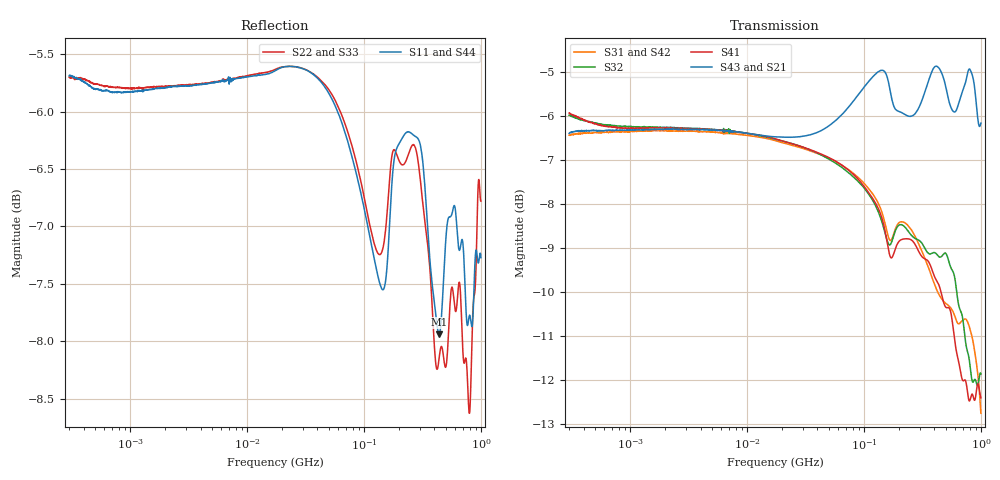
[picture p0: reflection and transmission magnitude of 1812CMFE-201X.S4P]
!s-Parameter Generated by FASTRON Sdn. Bhd.
!FASTRON P/N : 1812CMF/E-201X
!Keysight Technologies: E5071C_MY46733604_B.14.02
!Date: Mon Mar 09 11:25:32 2026
!Version  :Rev00  Mon Mar 09 11:25:32 2026
!Data & Calibration Information:
!Freq	S11:SOLT4(ON)	S12:SOLT4(ON)	S13:SOLT4(ON)	S14:SOLT4(ON)
!	S21:SOLT4(ON)	S22:SOLT4(ON)	S23:SOLT4(ON)	S24:SOLT4(ON)
!	S31:SOLT4(ON)	S32:SOLT4(ON)	S33:SOLT4(ON)	S34:SOLT4(ON)
!	S41:SOLT4(ON)	S42:SOLT4(ON)	S43:SOLT4(ON)	S44:SOLT4(ON)
!PortZ  Port1:50+j0  Port2:50+j0  Port3:50+j0  Port4:50+j0
!When reading reference impedance value at option line is always used.
! Remarks : This data is being provided solely for informational purposes.
# Hz S dB R 50
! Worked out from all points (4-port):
!   1601 points, 300 kHz to 1 GHz, reference 50 ohm
!   strongest paths, dB at 300 kHz, 2.303 MHz, 17.55 MHz, 132.8 MHz, 1 GHz:
!     S43: -6.4, -6.3, -6.5, -5.0, -6.2
!     S21: -6.5, -6.3, -6.5, -5.0, -6.1
!     S41: -5.9, -6.3, -6.5, -8.1, -12.4
!     S32: -6.0, -6.3, -6.5, -8.2, -11.9
!     S31: -6.4, -6.3, -6.6, -8.0, -12.8
!     S42: -6.4, -6.3, -6.6, -8.0, -13.3
!   lowest |S11| = -7.9 dB at 438.7 MHz (marker M1), VSWR 2.34, Z = 110 - j25 ohm
!   |S11| at or under -10 dB: nowhere
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300000  -5.69 6.9  -6.48 8.8  -6.45 -171.6  -6.04 -9.0
        -6.45 8.5  -5.70 7.4  -5.96 -9.2  -6.51 -171.5
        -6.44 -171.8  -5.98 -9.1  -5.69 7.2  -6.50 8.8
        -5.93 -9.4  -6.42 -171.8  -6.40 8.3  -5.79 7.9
2.707884e7  -5.61 -3.8  -6.49 1.9  -6.68 159.4  -6.68 -20.6
            -6.50 1.9  -5.61 -4.2  -6.66 -20.9  -6.72 159.1
            -6.70 159.3  -6.67 -21.0  -5.57 -4.0  -6.52 1.9
            -6.67 -20.6  -6.70 159.1  -6.47 1.8  -5.59 -3.8
1.235257e8  -7.30 -11.0  -5.07 0.1  -7.82 95.7  -7.95 -83.8
            -5.08 0.1  -7.16 -12.8  -7.99 -84.8  -7.87 95.1
            -7.84 95.6  -8.00 -84.8  -7.06 -13.9  -5.09 1.5
            -7.95 -83.9  -7.86 95.1  -5.06 1.4  -7.20 -13.0
2.744993e8  -6.21 -15.7  -6.02 -0.9  -8.72 9.1  -8.94 -171.4
            -6.03 -0.9  -6.31 -21.1  -8.78 -175.9  -8.73 8.4
            -8.75 9.2  -8.79 -175.8  -6.26 -20.1  -5.99 0.0
            -8.93 -171.5  -8.71 8.4  -5.94 0.0  -6.27 -17.3
4.386828e8  -7.94 -13.8  -5.01 -7.9  -10.04 -85.9  -9.85 92.3
            -5.02 -7.9  -8.15 -23.9  -9.21 89.0  -10.30 -87.7
            -10.07 -85.9  -9.20 89.0  -8.06 -22.7  -4.91 -5.5
            -9.86 92.3  -10.29 -87.6  -4.91 -5.6  -8.12 -20.1
7.352652e8  -7.58 -8.7  -5.38 -10.3  -10.60 103.3  -12.03 -75.8
            -5.39 -10.2  -8.15 -16.4  -11.09 -75.1  -10.65 100.2
            -10.62 103.5  -11.09 -74.9  -8.26 -15.4  -5.23 -6.2
            -12.01 -75.4  -10.64 100.5  -5.26 -6.2  -7.73 -16.4
1e9  -7.27 5.6  -6.13 -19.4  -12.76 -41.2  -12.40 123.2
     -6.15 -19.3  -6.78 -2.2  -11.89 130.6  -13.35 -41.8
     -12.77 -41.1  -11.87 130.8  -7.14 -2.6  -6.18 -11.1
     -12.42 122.9  -13.34 -41.6  -6.16 -10.9  -7.38 -9.1
